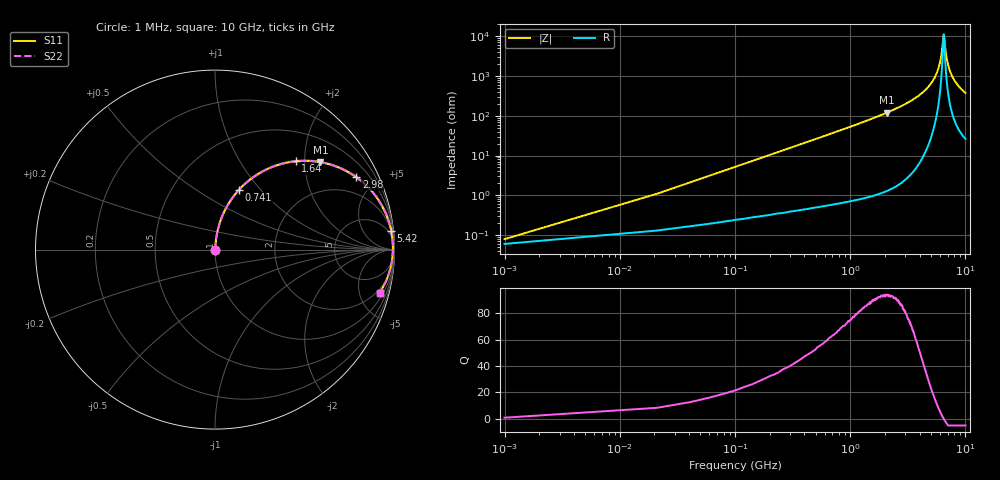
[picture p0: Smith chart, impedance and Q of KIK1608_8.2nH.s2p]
!version-2
!date-01.2022
!Series
# MHz S RI R 50
!Freq ReS11 ImS11 ReS21 ImS21 ReS12 ImS12 ReS22 ImS22
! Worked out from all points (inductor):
!   501 points, 1 MHz to 10 GHz, reference 50 ohm
!   read as one part in series: L = 8.2 nH near 41 MHz
!   highest Q = 93.5 at 2.08 GHz (marker M1), where L = 9.14 nH
!   self-resonance near 6.48 GHz
!   S11 on the Smith chart (normalised r, x): 1 MHz: 1.00, +0.00; 741 MHz: 1.01, +0.77; 1.64 GHz: 1.02, +1.81; 2.98 GHz: 1.05, +3.89; 5.42 GHz: 2, +18; 10 GHz: 1.53, -7.48
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1  0.000595 0.000515  0.9994 -0.000515  0.9994 -0.000515  0.000595 0.000515
61  0.00293 0.0313  0.9971 -0.0313  0.9971 -0.0313  0.00293 0.0313
101  0.00508 0.0517  0.9949 -0.0517  0.9949 -0.0517  0.00508 0.0517
161  0.0097 0.082  0.9903 -0.082  0.9903 -0.082  0.0097 0.082
381  0.0412 0.1881  0.9588 -0.1881  0.9588 -0.1881  0.0412 0.1881
741  0.134 0.333  0.866 -0.333  0.866 -0.333  0.134 0.333
1640  0.4499 0.492  0.5501 -0.492  0.5501 -0.492  0.4499 0.492
1680  0.4633 0.4932  0.5367 -0.4932  0.5367 -0.4932  0.4633 0.4932
2080  0.5873 0.487  0.4127 -0.487  0.4127 -0.487  0.5873 0.487
2980  0.7883 0.4024  0.2117 -0.4024  0.2117 -0.4024  0.7883 0.4024
3340  0.8424 0.3575  0.1576 -0.3575  0.1576 -0.3575  0.8424 0.3575
5020  0.9703 0.1496  0.0297 -0.1496  0.0297 -0.1496  0.9703 0.1496
5420  0.9815 0.1055  0.0185 -0.1055  0.0185 -0.1055  0.9815 0.1055
6060  0.9902 0.0402  0.00977 -0.0402  0.00977 -0.0402  0.9902 0.0402
6240  0.991 0.0231  0.00899 -0.0231  0.00899 -0.0231  0.991 0.0231
6480  0.9911 0.000878  0.00891 -0.000878  0.00891 -0.000878  0.9911 0.000878
6540  0.9909 -0.00453  0.00905 0.00453  0.00905 0.00453  0.9909 -0.00453
6680  0.9904 -0.0169  0.00961 0.0169  0.00961 0.0169  0.9904 -0.0169
6920  0.9887 -0.0376  0.0112 0.0376  0.0112 0.0376  0.9887 -0.0376
7240  0.9853 -0.0639  0.0147 0.0639  0.0147 0.0639  0.9853 -0.0639
8340  0.9651 -0.1442  0.0349 0.1442  0.0349 0.1442  0.9651 -0.1442
10000  0.9189 -0.2401  0.0811 0.2401  0.0811 0.2401  0.9189 -0.2401
